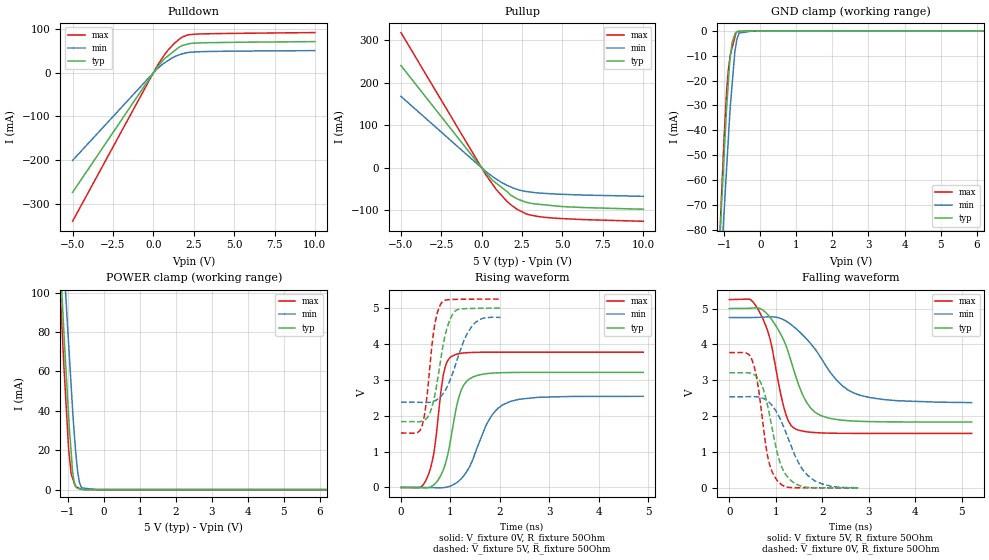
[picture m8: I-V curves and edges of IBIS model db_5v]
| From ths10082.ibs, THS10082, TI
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|   db_5v Model
[Model]   db_5v
Model_type   I/O
Polarity   Non-Inverting
Enable   Active-High
Vinl = 0.6
Vinh = 2.6
Vmeas = 2.5
Vref = 2.5
Cref = 30pF
Rref = 50
|   typ   min   max
C_comp   1.730e-12   1.724e-12   1.754e-12
[Voltage Range]   5   4.75   5.25
|Ambient Temperature   25   85   -40
|Junction Temperature
[Temperature Range]   27   125   -40
[Pullup Reference]   5   4.75   5.25
[Pulldown Reference]   0   0   0
[Power Clamp Reference]   5   4.75   5.25
[GND Clamp Reference]   0   0   0
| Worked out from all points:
|   slope of the pulldown table from 0 to 0.75 V, typ, clamps not added: 21.9 ohm
|   slope of the pullup table from 0 to 0.75 V, typ, clamps not added: 23.7 ohm
|   GND clamp passes 1 mA (typ) near -0.70 V on its own axis
|   POWER clamp passes 1 mA (typ) near -0.76 V on its own axis
|   falling waveform, V_fixture 5V, R_fixture 50Ohm: 20-80 % time 556ps typ, 858ps min, 381ps max; typ from 5 V to 1.84 V
|   rising waveform, V_fixture 0V, R_fixture 50Ohm: 20-80 % time 288ps typ, 492ps min, 207ps max; typ from 0 V to 3.21 V
|   rising waveform, V_fixture 5V, R_fixture 50Ohm: 20-80 % time 248ps typ, 384ps min, 178ps max; typ from 1.84 V to 5 V
|   falling waveform, V_fixture 0V, R_fixture 50Ohm: 20-80 % time 337ps typ, 526ps min, 250ps max; typ from 3.21 V to 0 V
[Pulldown]
|   Voltage   I(typ)   I(min)   I(max)
-5V       -273.8mA   -200.7mA   -340.2mA
278.2mV   14.45mA    10.34mA    18.49mA
700mV     32.81mA    23.07mA    41.84mA
924mV     39.34mA    28.46mA    52.67mA
1.292V    50.04mA    36.47mA    67.25mA
1.596V    58.91mA    41.32mA    76.89mA
1.848V    63.09mA    44.11mA    83.04mA
2.142V    65.97mA    46.51mA    87mA
2.635V    68.25mA    47.94mA    88.77mA
10V       71.52mA    50.93mA    92.28mA
[GND Clamp]
|   Voltage   I(typ)   I(min)   I(max)
-5V       -1.585A    -1.476A    -1.708A
-1.306V   -142mA     -156.3mA   -147.7mA
-1.088V   -72.58mA   -93.58mA   -68.81mA
-1.04V    -59.06mA   -80.67mA   -53.32mA
-1.003V   -48.54mA   -71.33mA   -41.37mA
-934.5mV  -30.27mA   -54.33mA   -23.53mA
-840mV    -10.75mA   -31.23mA   -9.866mA
-785mV    -4.643mA   -21.48mA   -6.793mA
-712.5mV  -1.61mA    -8.842mA   -2.741mA
-640mV    -254uA     -2.942mA   -291uA
-190mV    0A         -26.17nA   -86.38uA
10V       0A         0A         0A
[Pullup]
|   Voltage   I(typ)   I(min)   I(max)
-5V       240.8mA    168.3mA    318.4mA
288.8mV   -13.19mA   -9.295mA   -17.98mA
700mV     -30.18mA   -21.2mA    -40.11mA
924mV     -36.77mA   -26.8mA    -51.95mA
1.533V    -54.69mA   -40.35mA   -77.44mA
1.822V    -64.84mA   -45.16mA   -87.17mA
2.2V      -72.69mA   -50.69mA   -97.65mA
2.751V    -80.58mA   -55.49mA   -108.1mA
3.838V    -86.66mA   -59.79mA   -115.9mA
5.405V    -91.76mA   -62.72mA   -120mA
10V       -97.14mA   -66.87mA   -125.6mA
[POWER Clamp]
|   Voltage   I(typ)   I(min)   I(max)
-5V       1.658A     1.635A     1.693A
-1.306V   151.2mA    185.3mA    137.9mA
-1.103V   79.28mA    115.5mA    62mA
-1.08V    71.42mA    107.8mA    54.79mA
-1.026V   54.28mA    90.08mA    37.5mA
-971.2mV  36.91mA    73.49mA    20.28mA
-903mV    19.05mA    52.81mA    7.974mA
-855mV    8.079mA    38.27mA    5.384mA
-815mV    3.446mA    28.17mA    3.226mA
-726.8mV  728.7uA    9.767mA    1.096mA
-640mV    112.2uA    2.129mA    234.5uA
10V       0A         0A         0A
[Ramp]
R_load = 50
|   typ   min   max
dV/dt_r   1.92515/2.85986e-10   1.52416/4.90559e-10   2.26293/2.06457e-10
dV/dt_f   1.89784/5.54728e-10   1.42308/8.57426e-10   2.23898/3.79943e-10
[Falling Waveform]
V_fixture = 5V
V_fixture_min = 4.75V
V_fixture_max = 5.25V
R_fixture = 50Ohm
|   Time   V(typ)   V(min)   V(max)
0s        5V         4.75V      5.25V
438ps     5.007V     4.749V     5.262V
652ps     5.006V     4.756V     4.898V
876ps     4.754V     4.769V     4.153V
1.2ns     4.028V     4.665V     2.124V
1.402ns   3.22V      4.476V     1.658V
1.832ns   2.121V     3.889V     1.543V
2.296ns   1.908V     3.02V      1.523V
2.676ns   1.863V     2.645V     1.519V
5.212ns   1.837V     2.378V     1.518V
[Rising Waveform]
V_fixture = 0V
V_fixture_min = 0V
V_fixture_max = 0V
R_fixture = 50Ohm
|   Time   V(typ)   V(min)   V(max)
0s        1.848nV    2.664nV    1.618nV
550ps     -5.442mV   -2.645mV   340.9mV
672ps     82.34mV    -6.578mV   1.022V
862ps     511.8mV    -4.324mV   3.168V
1.03ns    1.545V     56.11mV    3.659V
1.164ns   2.483V     172.9mV    3.726V
1.33ns    2.961V     443mV      3.756V
1.76ns    3.176V     1.834V     3.77V
2.066ns   3.2V       2.31V      3.771V
4.898ns   3.209V     2.54V      3.772V
[Rising Waveform]
V_fixture = 5V
V_fixture_min = 4.75V
V_fixture_max = 5.25V
R_fixture = 50Ohm
|   Time   V(typ)   V(min)   V(max)
0s        1.837V     2.378V     1.518V
424ps     1.846V     2.37V      1.706V
510ps     1.913V     2.367V     2.352V
684ps     2.569V     2.415V     4.543V
826ps     3.764V     2.566V     5.157V
934ps     4.459V     2.806V     5.23V
1.094ns   4.912V     3.379V     5.242V
1.296ns   4.983V     4.165V     5.248V
1.486ns   4.991V     4.574V     5.249V
2.014ns   4.999V     4.74V      5.25V
[Falling Waveform]
V_fixture = 0V
V_fixture_min = 0V
V_fixture_max = 0V
R_fixture = 50Ohm
|   Time   V(typ)   V(min)   V(max)
0s        3.209V     2.54V      3.772V
488ps     3.186V     2.544V     3.565V
612ps     3.068V     2.537V     2.895V
738ps     2.724V     2.491V     1.643V
842ps     2.177V     2.402V     777mV
1.066ns   810.8mV    1.997V     152.9mV
1.31ns    222.8mV    1.235V     8.754mV
1.684ns   12.44mV    349.1mV    1.566mV
2.168ns   2.045mV    52mV       371.5uV
2.784ns   453.1uV    3.45mV     196.1uV
